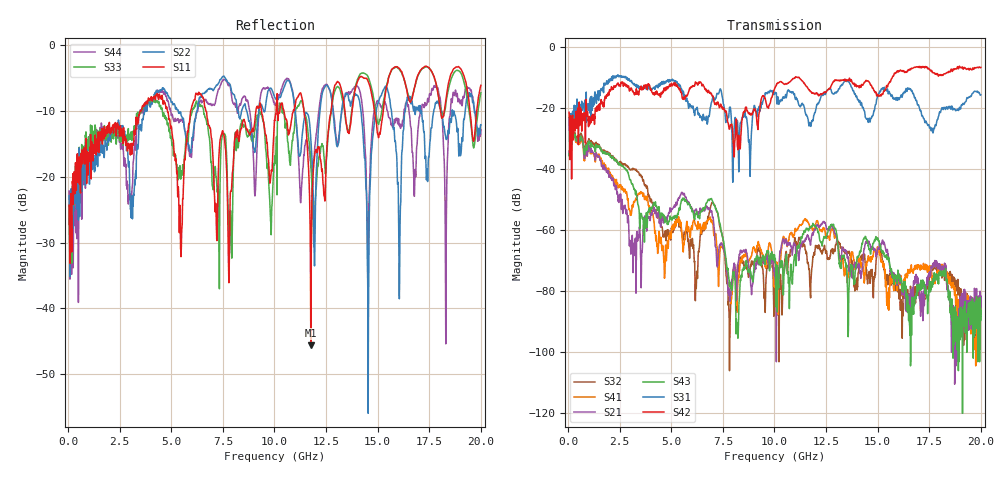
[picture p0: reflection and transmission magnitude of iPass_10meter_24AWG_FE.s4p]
! FILE: D:\iPass\iPassCables1205\10meter\iPass_10meter_24AWG_FE.s4p
# MHz S MA R 50.00
! FREQ  S11  S12  S13  S14
!  S21  S22  S23  S24
!  S31  S32  S33  S34
!  S41  S42  S43  S44
!  MAG  ANG  MAG  ANG  MAG  ANG  MAG  ANG
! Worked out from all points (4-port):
!   1996 points, 50 MHz to 20 GHz, reference 50 ohm
!   strongest paths, dB at 50 MHz, 5.04 GHz, 10.03 GHz, 15.02 GHz, 20 GHz:
!     S42: -21.3, -12.6, -13.2, -15.9, -6.7
!     S31: -23.2, -10.6, -14.8, -15.6, -15.6
!     S43: -35.0, -56.6, -69.3, -63.2, -85.7
!     S21: -34.1, -53.2, -75.8, -66.1, -81.5
!     S41: -33.9, -58.7, -74.7, -66.6, -87.3
!     S32: -34.9, -59.0, -77.1, -66.2, -81.9
!   lowest |S11| = -45.6 dB at 11.76 GHz (marker M1), VSWR 1.01, Z = 49.5 - j0.227 ohm
!   |S11| at or under -10 dB: start of sweep to 3.521 GHz; 6.679 GHz to 9.1 GHz (2.422 GHz wide, 30.7 % of centre); 11.43 GHz to 12.74 GHz (1.314 GHz wide, 10.9 % of centre)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
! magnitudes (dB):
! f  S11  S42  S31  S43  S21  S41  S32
! 50 MHz  -24.3  -21.3  -23.2  -35.0  -34.1  -33.9  -34.9
! 3.22 GHz  -13.3  -15.6  -12.1  -46.7  -66.2  -50.6  -39.9
! 6.21 GHz  -7.3  -11.9  -20.1  -54.2  -53.0  -58.8  -79.1
! 7.04 GHz  -18.5  -16.6  -16.5  -51.4  -56.7  -59.9  -51.1
! 7.85 GHz  -23.5  -26.0  -19.6  -78.5  -83.2  -82.7  -89.6
! 11.76 GHz  -45.6  -14.6  -26.0  -59.2  -63.9  -59.3  -77.4
! 20 GHz  -6.1  -6.7  -15.6  -85.7  -81.5  -87.3  -81.9
